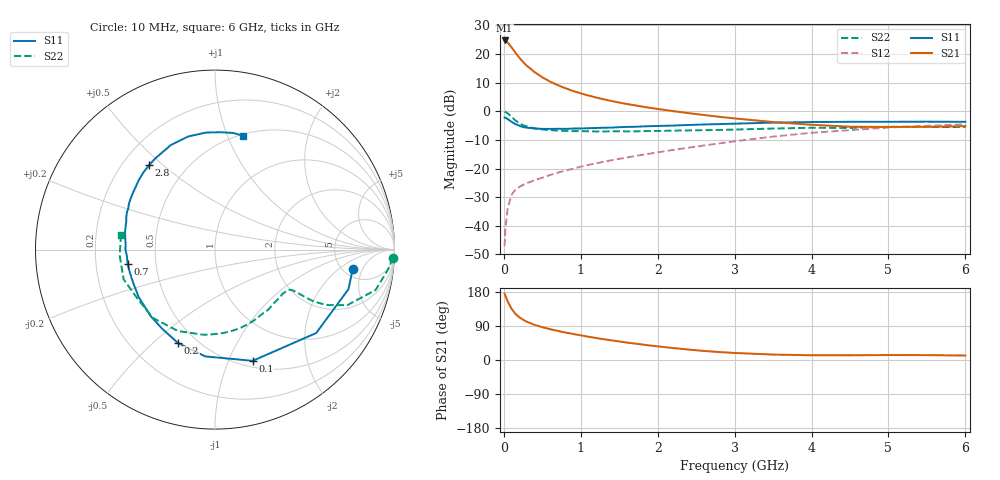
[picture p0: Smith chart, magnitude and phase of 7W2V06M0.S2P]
! Infineon Technologies  Discrete & RF Semiconductors
! BFS17W
! Si NPN RF Bipolar Junction Transistor in SOT323
! VCE = 2 V  IC = 6 mA
! Common Emitter S-Parameters:  August  1999
# GHz  S  MA  R  50
!  f  S11  S21  S12  S22
! GHz  MAG  ANG  MAG  ANG  MAG  ANG  MAG  ANG
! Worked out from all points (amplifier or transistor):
!   36 points, 10 MHz to 6 GHz, reference 50 ohm
!   highest |S21| = 24.7 dB at 10 MHz (marker M1)
!   |S21| within 3 dB of that: start of sweep to 116 MHz
!   unconditionally stable (mu >= 1): 483.3 MHz to 3.256 GHz; 3.872 GHz to end of sweep
!   at 250 MHz: K = 0.66, MSG = 21.5 dB, |S12| = -25.7 dB
!   at 1.4 GHz: K = 1.27, MAG = 7.2 dB, |S12| = -17.1 dB
!   at 6 GHz: K = 1.10, MAG = -2.2 dB, |S12| = -4.6 dB
!   S11 on the Smith chart (normalised r, x): 10 MHz: 6.04, -3.30; 100 MHz: 0.57, -1.23; 200 MHz: 0.40, -0.60; 700 MHz: 0.34, -0.07; 2.8 GHz: 0.31, +0.45; 6 GHz: 0.51, +1.14
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0.01  0.7749 -8.1  17.23 175.2  0.0044 86.0  0.9911 -2.6
0.02  0.7757 -16.5  17.07 169.4  0.0087 80.8  0.9741 -6.1
0.05  0.7308 -39.5  15.9 154.5  0.0204 72.4  0.9227 -14.1
0.1  0.6543 -71.3  13.06 135.4  0.0347 58.8  0.7995 -22.8
0.15  0.5975 -95.3  10.56 122.0  0.0425 52.6  0.6918 -26.5
0.2  0.5599 -111.6  8.668 112.9  0.0476 49.5  0.621 -27.7
0.25  0.5295 -124.1  7.257 106.2  0.0517 47.4  0.5712 -27.8
0.3  0.5156 -134.0  6.223 100.9  0.0555 47.9  0.5407 -27.7
0.4  0.5007 -148.1  4.818 92.7  0.0627 49.4  0.5003 -27.6
0.5  0.4921 -157.8  3.92 86.6  0.069 51.5  0.4805 -27.8
0.6  0.4913 -164.9  3.296 81.4  0.0769 53.5  0.4678 -28.7
0.7  0.4936 -170.8  2.862 76.8  0.0845 55.2  0.4597 -30.1
0.9  0.4989 -180.0  2.26 68.7  0.099 58.0  0.4491 -33.8
1.1  0.5054 172.0  1.881 61.4  0.1156 59.3  0.4464 -38.6
1.3  0.515 165.3  1.616 54.8  0.1315 60.4  0.4433 -44.0
1.6  0.5331 156.9  1.336 46.0  0.1557 61.7  0.4442 -52.4
2.2  0.5623 142.1  1.006 31.5  0.2106 62.6  0.4582 -71.2
2.8  0.5966 127.9  0.8 21.0  0.2744 60.9  0.4716 -91.0
3.5  0.6327 112.8  0.648 14.3  0.361 55.8  0.4983 -114.3
4.5  0.654 94.4  0.537 12.4  0.4679 43.8  0.5115 -148.2
5.5  0.6578 81.2  0.535 12.9  0.5564 31.8  0.532 -176.3
6  0.6538 76.2  0.55 11.8  0.5907 26.0  0.53 171.4
